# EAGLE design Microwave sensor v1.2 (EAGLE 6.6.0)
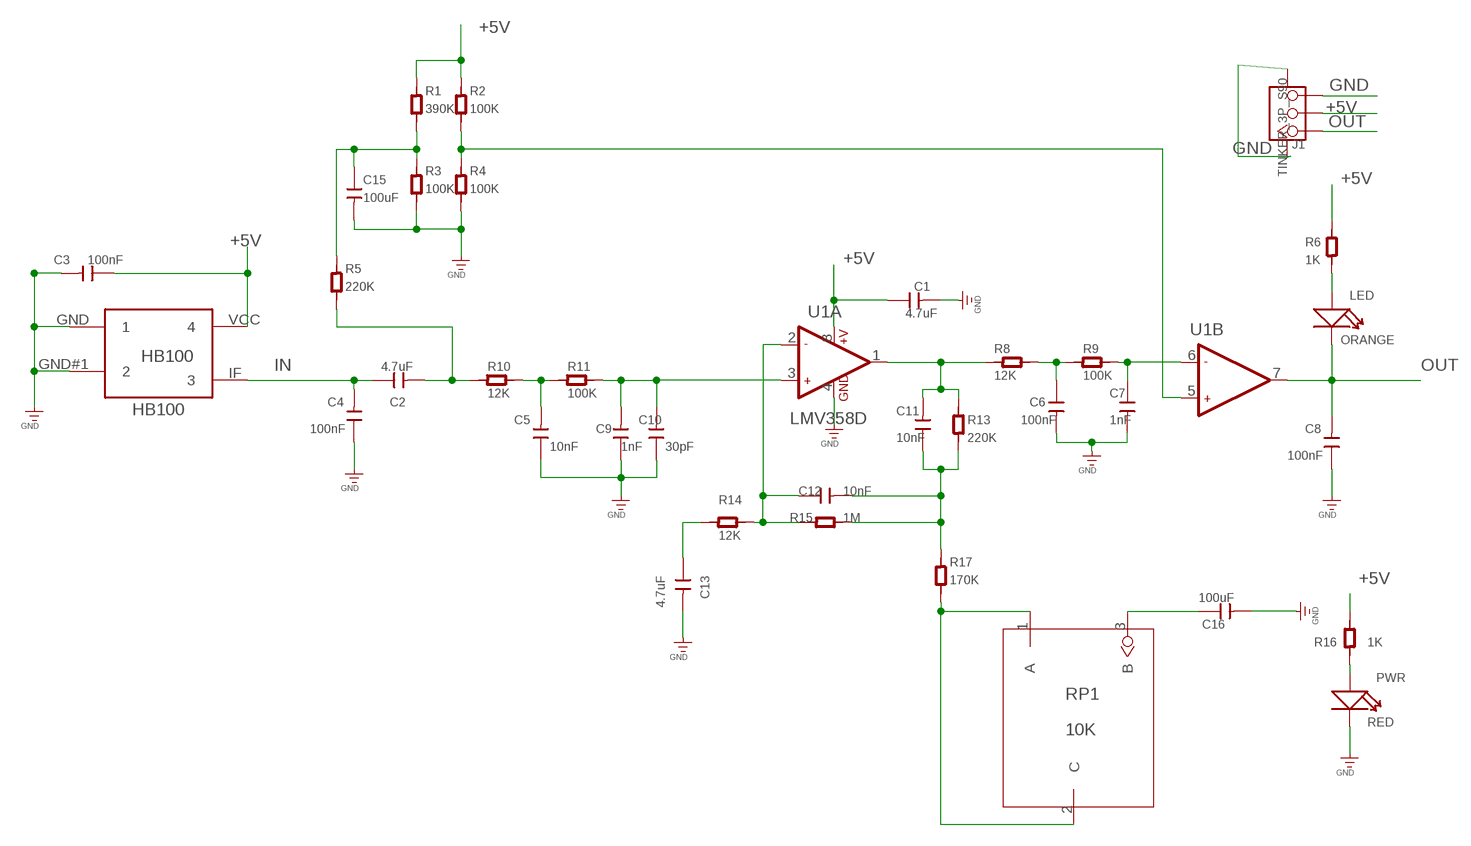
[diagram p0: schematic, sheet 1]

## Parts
C1  4.7uF  C-0603  [C0603]
C2  4.7uF  C-0603  [C0603]
C3  100nF  C-0603  [C0603]
C4  100nF  C-0603  [C0603]
C5  10nF  C-0603  [C0603]
C6  100nF  C-0603  [C0603]
C7  1nF  C-0603  [C0603]
C8  100nF  C-0603  [C0603]
C9  1nF  C-0603  [C0603]
C10  30pF  C-0603  [C0603]
C11  10nF  C-0603  [C0603]
C12  10nF  C-0603  [C0603]
C13  4.7uF  C-0603  [C0603]
C15  100uF  C-1210  [C1210]
C16  100uF  C-1210  [C1210]
HB100  MICROWAVE  [MICROWAVE]
J1  TINKER_3P_S90  [TINKER_3P_S90]
LED  ORANGE  LED'0805'  [LED-0805]
PWR  RED  LED'0805'  [LED-0805]
R1  390K  R-0603  [R0603]
R2  100K  R-0603  [R0603]
R3  100K  R-0603  [R0603]
R4  100K  R-0603  [R0603]
R5  220K  R-0603  [R0603]
R6  1K  R-0603  [R0603]
R8  12K  R-0603  [R0603]
R9  100K  R-0603  [R0603]
R10  12K  R-0603  [R0603]
R11  100K  R-0603  [R0603]
R13  220K  R-0603  [R0603]
R14  12K  R-0603  [R0603]
R15  1M  R-0603  [R0603]
R16  1K  R-0603  [R0603]
R17  170K  R-0603  [R0603]
RP1  10K  DEVICE_RESISTANCE  [PACKAGE__RESISTANCE]
U1  LMV358D  [SO08]

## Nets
+5V: C1.1 C3.1 HB100.VCC J1.2 R1.1 R2.1 R6.2 R16.2 U1.8(A:+V)
GND: C1.2 C3.2 C4.1 C5.1 C6.2 C7.2 C8.1 C9.1 C10.1 C13.2 C15.2 C16.2 HB100.GND HB100.GND#1 J1.3 J1.SS1 J1.SS2 PWR.- R3.2 R4.2 U1.4(A:GND)
IN: C2.1 C4.2 HB100.IF
N$1: C15.1 R1.2 R3.1 R5.1
N$3: C6.1 R8.2 R9.1
N$4: R2.2 R4.1 U1.5(B:+IN2)
N$5: C13.1 R14.1
N$6: C2.2 R5.2 R10.1
N$7: C11.1 C12.2 R13.1 R15.2 R17.1
N$8: C5.2 R10.2 R11.1
N$9: C11.2 R8.1 R13.2 U1.1(A:OUT1)
N$10: C9.2 C10.2 R11.2 U1.3(A:+IN1)
N$11: C7.1 R9.2 U1.6(B:-IN2)
N$12: C12.1 R14.2 R15.1 U1.2(A:-IN1)
N$13: R17.2 RP1.1(A) RP1.2(C)
N$14: C16.1 RP1.3(B)
N$16: PWR.+ R16.1
N$17: LED.+ R6.1
OUT: C8.2 J1.1 LED.- U1.7(B:OUT2)

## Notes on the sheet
- HB100

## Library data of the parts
C1-C13 C15 C16 = Discrete:C*: Ceramic Capacitors
HB100 = Microwave:MICROWAVE
J1 = Connector:TINKER_3P_S90
LED PWR = Discrete:LED*
R1-R6 R8-R11 R13-R17 = OPL Eagle Library:R*
RP1 = test:DEVICE_RESISTANCE
U1 = IC:LMV358: General purpose LOW Voltage, Rail-to-Rail Output Amplifiers http://www.fairchildsemi.com/ds/LM/LMV358.pdf

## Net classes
0 default: width 0.152 mm, drill 0.305 mm, clearance 0.152 mm

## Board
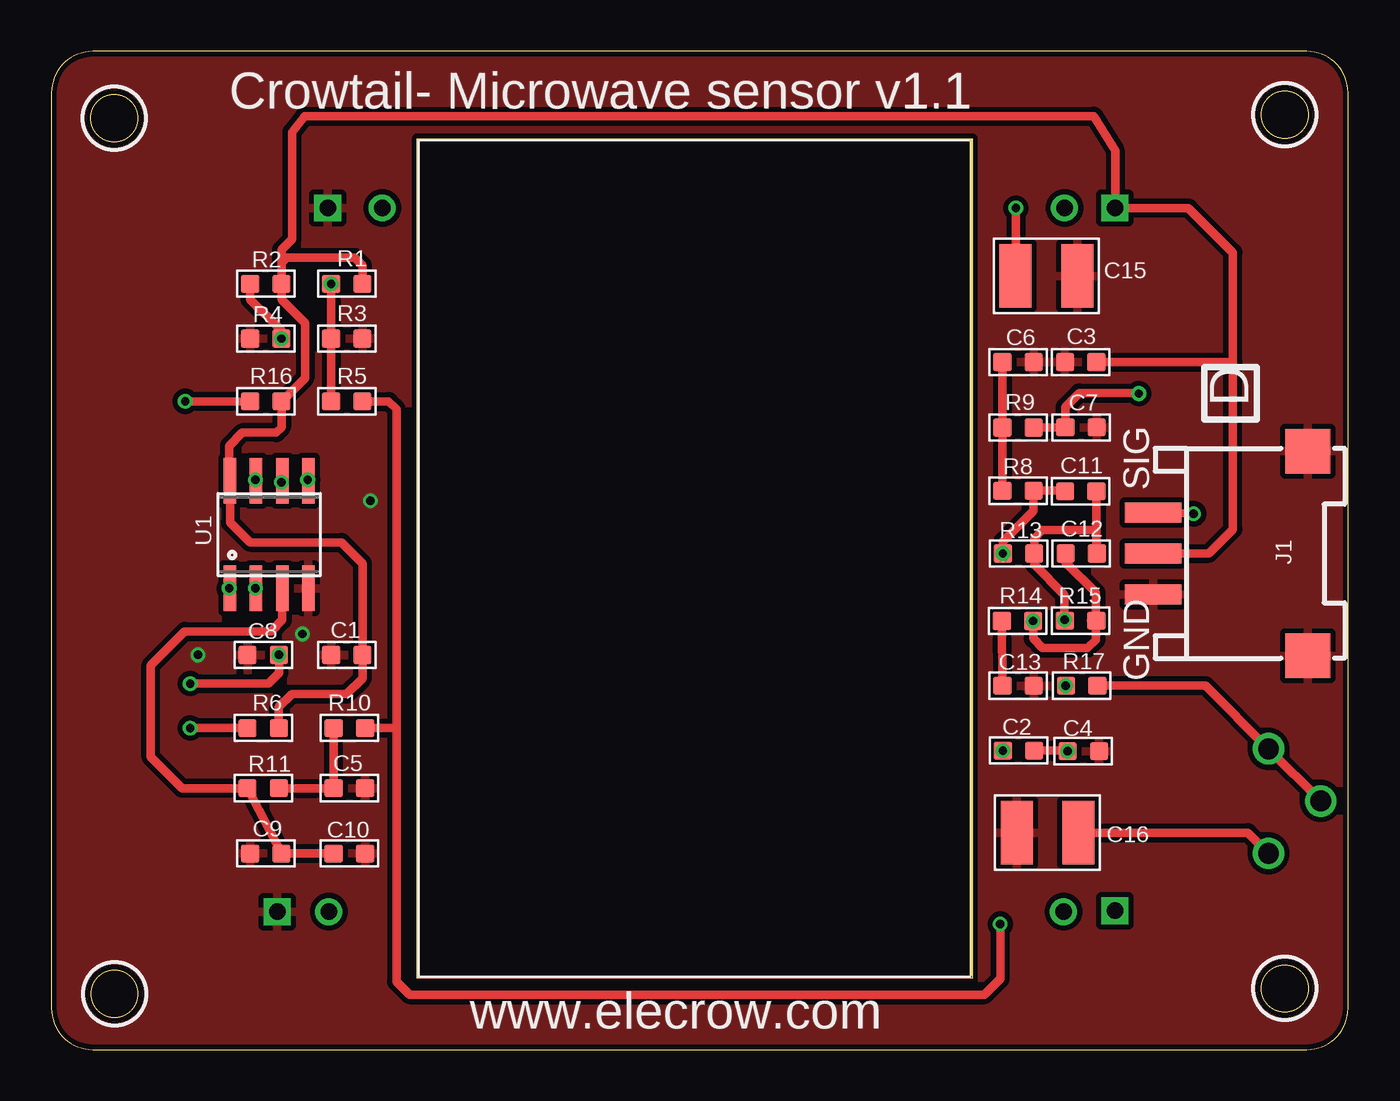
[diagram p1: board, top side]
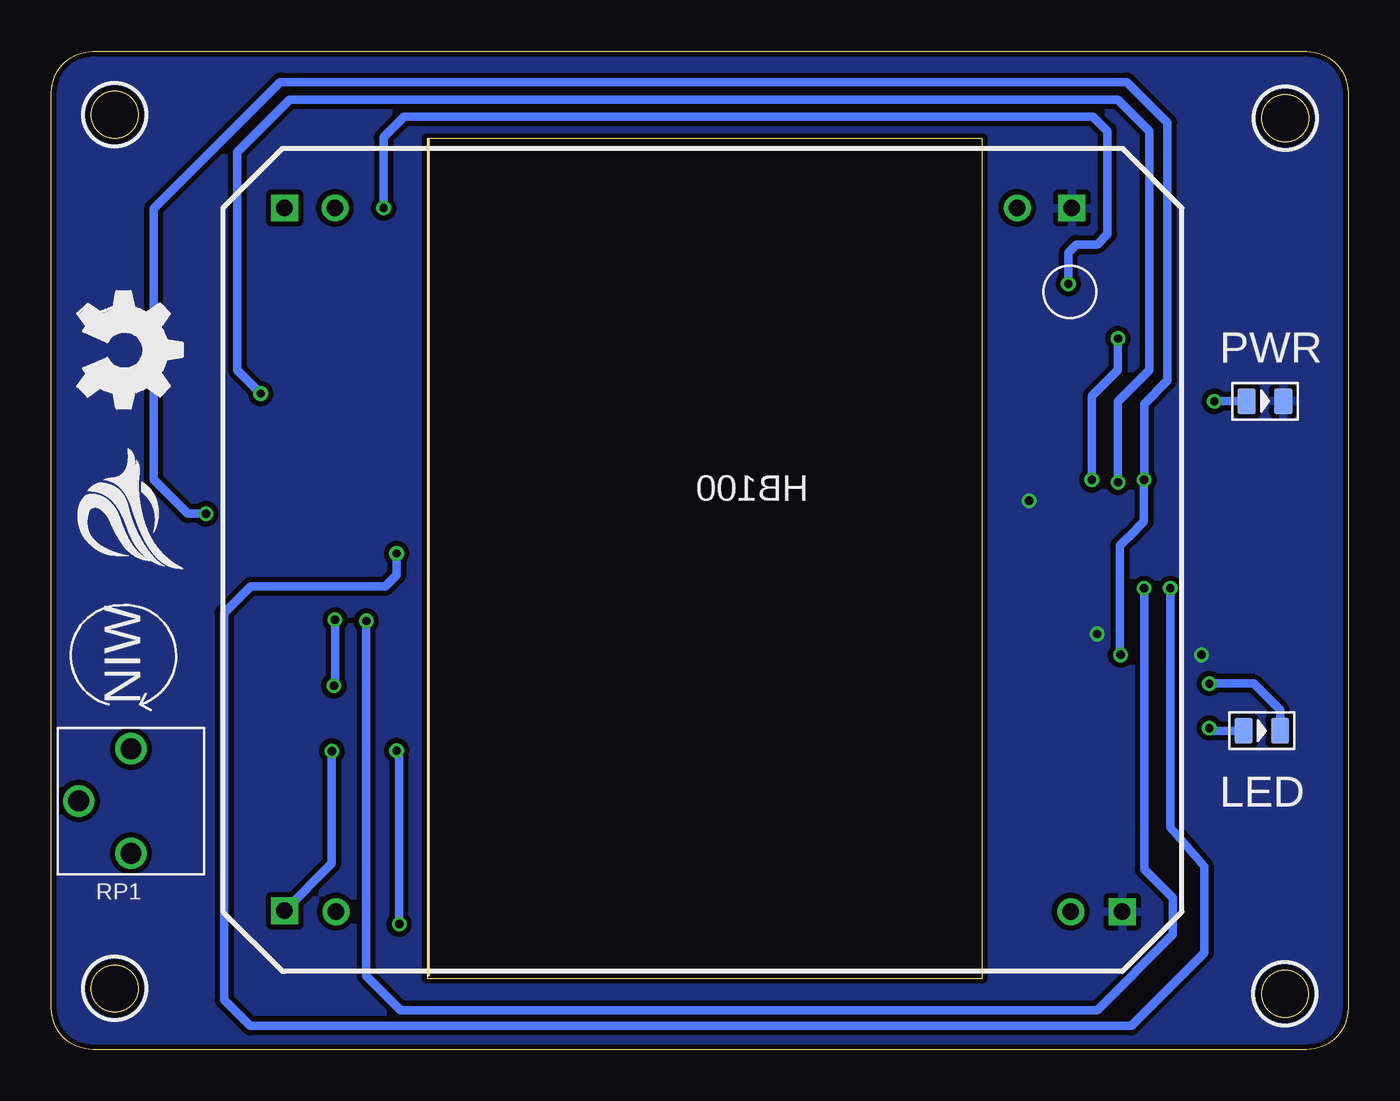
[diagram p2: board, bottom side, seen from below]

Size 63 x 48.5 mm. Coordinates in mm from the lower left corner, seen from the top.
Outline: 0,46.5 0,2 arc90 2,0 61,0 arc90 63,2 63,46.5 arc90 61,48.5 2,48.5 arc90 0,46.5
Outline: 17.75,44.27 44.76,44.27 44.76,3.45 17.75,3.45 17.75,44.27
Outline: circle at 3.06,2.71 radius 1.14
Outline: circle at 3.05,45.26 radius 1.14
Outline: circle at 59.92,45.42 radius 1.14
Outline: circle at 59.92,2.97 radius 1.14
Copper layers (1*16): Top 0.035mm / dielectric 1.5mm / Bottom 0.035mm
Design rules: minimum track width 6mil, minimum drill 12mil, track to track 6mil, track to pad 6mil, pad to pad 6mil, via to via 6mil, smd to smd 0mil, copper to edge 10mil, drill to drill 10mil, minimum pad ring 10mil, minimum via ring 6mil, stop-mask expansion 2mil, vias tented up to drill 100mil, thermal gap 10mil

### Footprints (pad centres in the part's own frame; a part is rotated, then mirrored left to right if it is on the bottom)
C0603 = smd 0.889 x 0.889: 1 -0.762,0; 2 0.762,0
C1210 = smd 1.55 x 3.1: 1 -1.5,0; 2 1.5,0
MICROWAVE = drill 0.8 square: GND 2.45,37.1; GND#1 0,2.9; IF 40.7,2.95; VCC 40.7,37.1 | drill 0.8: P$2 2.5,2.9; P$4 38.2,2.9; P$6 5.1,37.1; P$8 38.25,37.1
TINKER_3P_S90 = smd 0.965 x 2.74: 1 -1.984,-4.545; 2 0.016,-4.545; 3 2.016,-4.545 | smd 2.159 x 2.184: SS1 -4.958,2.955; SS2 4.99,2.955
LED-0805 = smd 0.889 x 1.27: + -0.889,0; - 0.889,0
R0603 = smd 0.889 x 0.889: 1 -0.762,0; 2 0.762,0
PACKAGE__RESISTANCE = drill 1.016: 1 -2.286,-0.254; 2 0.254,-2.794; 3 2.794,-0.254
SO08 = smd 0.61 x 2.21: 1 -1.905,-2.616; 2 -0.635,-2.616; 3 0.635,-2.616; 4 1.905,-2.616; 5 1.905,2.616; 6 0.635,2.616; 7 -0.635,2.616; 8 -1.905,2.616

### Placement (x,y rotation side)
C1  14.35,19.18 180 top
C2  46.99,14.53 180 top
C3  50.01,33.4 180 top
C4  50.14,14.5 180 top
C5  14.48,12.7 180 top
C6  46.96,33.4 0 top
C7  50.02,30.23 0 top
C8  10.29,19.18 0 top
C9  10.41,9.53 0 top
C10  14.48,9.53 180 top
C11  50.01,27.13 180 top
C12  50.04,24.1 0 top
C13  46.96,17.68 0 top
C15  48.35,37.59 0 top
C16  48.4,10.54 180 top
HB100  10.98,3.8 0 top
J1  58.08,24.12 270 top
LED  4.19,15.49 0 bottom
PWR  4.04,31.5 0 bottom
R1  14.35,37.21 180 top
R2  10.41,37.21 180 top
R3  14.35,34.54 0 top
R4  10.41,34.54 180 top
R5  14.35,31.5 0 top
R6  10.29,15.62 0 top
R8  46.96,27.15 180 top
R9  46.96,30.23 0 top
R10  14.48,15.62 180 top
R11  10.29,12.7 180 top
R13  46.99,24.1 180 top
R14  46.94,20.83 0 top
R15  50,20.83 180 top
R16  10.41,31.5 0 top
R17  50.06,17.68 0 top
RP1  58.88,12.33 270 bottom
U1  10.58,25.03 0 top
U$13  [ELECROW_NEW_4]  61.73,29.21 270 bottom
U$14  [OSHW_FILLX200_NOTEXT]  61.73,36.83 270 bottom
U$16  [MINIMUM]  63,16.51 0 bottom

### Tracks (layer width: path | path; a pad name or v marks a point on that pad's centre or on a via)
+5V
  Top 0.406: C3.1 57.4,33.4 | 11.18,38.23 R2.1 11.18,36.45 12.32,35.31 12.32,32.64 R16.2 11.18,30.23 10.92,29.97 9.27,29.97 8.64,29.34 8.64,27.68 U1.8 8.67,25.62 9.65,24.64 14.1,24.64 15.11,23.62 C1.1 15.11,18.03 14.35,17.27 11.68,17.27 11.05,16.64 R6.2 | 11.18,38.23 11.18,38.86 11.68,39.37 11.68,44.58 12.29,45.36 50.65,45.36 51.69,43.69 HB100.VCC 55.24,40.89 57.4,38.73 57.4,33.4 | R1.1 15.11,38.1 14.73,38.48 11.43,38.48 11.18,38.23 | J1.2 56.23,24.1 57.4,25.27 57.4,33.4
GND  (via drill 0.41)
  other vias: 15.49,26.67 12.19,20.19 7.11,19.18
  pour Bottom (isolate 0.254): -0.38,49.02 63.5,49.02 63.5,-0.38 -0.38,-0.38
  pour Top (isolate 0.254): -0.38,49.02 63.5,49.02 63.5,-0.38 -0.38,-0.38
IN  (via drill 0.41)
  Top 0.406: C2.1 49.34,14.53 C4.2
  Bottom 0.406: C4.2 49.38,9.05 HB100.IF
  other vias: 49.37,14.5
N$1  (via drill 0.41)
  Top 0.406: v46.86,40.89 46.86,37.61 C15.1 | R1.2 R3.1 R5.1
  Bottom 0.406: R1.2 13.59,38.73 13.21,39.12 12.19,39.12 11.68,39.62 11.68,44.63 12.39,45.34 45.85,45.34 46.86,44.33 v46.86,40.89
  other vias: 13.59,37.21
N$3
  Top 0.406: C6.1 R9.1 R8.2
N$4  (via drill 0.41)
  Top 0.406: R4.1 11.18,34.92 9.65,36.45 R2.2 | v12.45,27.69 v12.45,27.68 U1.5
  Bottom 0.406: R4.1 11.18,33.02 12.45,31.75 v12.45,27.69
  other vias: 11.18,34.54
N$5
  Top 0.406: R14.1 C13.1
N$6  (via drill 0.41)
  Top 0.406: R5.2 16.38,31.5 16.76,31.11 16.76,15.62 | 16.76,15.62 16.76,3.3 17.4,2.67 45.34,2.67 46.1,3.43 v46.1,6.1 | R10.1 16.76,15.62
  Bottom 0.406: v46.1,6.1 46.1,14.22 C2.2
  other vias: 46.23,14.53
N$7  (via drill 0.41)
  Top 0.406: R15.2 v49.23,20.88 49.23,22.1 47.75,23.57 R13.1 47.75,24.84 48.16,25.25 50.77,25.25 | R17.1 v49.28,17.68 49.28,17.73 | C11.1 50.77,25.25 | 50.77,25.25 50.77,24.13 C12.2 50.8,24.59
  Bottom 0.406: v49.23,20.88 49.23,17.73 v49.28,17.68
N$8
  Top 0.406: R11.1 C5.2 R10.2
N$9  (via drill 0.41)
  Top 0.406: C11.2 49,27.15 R8.1 47.7,27.13 47.7,26.16 46.23,24.69 R13.2 | U1.1 v8.64,22.41
  Bottom 0.406: v8.64,22.41 8.64,10.79 6.99,8.89 6.99,4.7 10.54,1.14 53.34,1.14 54.61,2.41 54.61,21.21 53.31,22.5 46.79,22.5 46.23,23.06 R13.2
  other vias: 46.23,24.1
N$10
  Top 0.406: U1.3 11.21,20.86 10.67,20.32 6.48,20.32 4.83,18.67 4.83,14.22 6.35,12.7 R11.2 C9.2 C10.2
N$11  (via drill 0.41)
  Top 0.406: U1.6 v11.18,27.56 | 49.02,30.32 C7.1 | R9.2 C7.1 | C7.1 49.26,31.23 49.94,31.9 52.81,31.9 v52.83,31.88
  Bottom 0.406: v11.18,27.56 11.18,31.5 9.65,33.02 9.65,44.63 11.18,46.15 51.44,46.15 53.98,43.61 53.98,33.02 v52.83,31.88
N$12  (via drill 0.41)
  Top 0.406: U1.2 v9.91,22.41 | 50.52,20.82 R15.1 | 50.49,20.85 R15.1 | R14.2 47.7,19.96 48.16,19.51 50.34,19.51 50.75,19.91 50.75,20.82 R15.1 | C12.1 49.28,23.67 50.75,22.2 50.75,20.85 R15.1
  Bottom 0.406: v9.91,22.41 9.91,8.76 8.51,7.37 8.51,5.59 12.19,1.91 46.02,1.91 47.7,3.58 R14.2
  other vias: 47.7,20.83
N$13
  Top 0.406: R17.2 56.07,17.68 RP1.1 RP1.2
N$14
  Top 0.406: C16.1 58.13,10.54 RP1.3
N$16  (via drill 0.41)
  Top 0.406: R16.1 v6.5,31.5
  Bottom 0.406: v6.5,31.5 PWR.+
N$17  (via drill 0.41)
  Top 0.406: R6.1 v6.74,15.62
  Bottom 0.406: LED.+ 6.74,15.49 v6.74,15.62
OUT  (via drill 0.41)
  Top 0.406: U1.7 v9.91,27.69 | J1.1 v55.5,26.04 | v6.74,17.78 10.55,17.78 11.06,18.29 C8.2
  Bottom 0.406: v55.5,26.04 56.39,26.04 58.04,27.69 58.04,40.87 51.89,47.02 10.74,47.02 8.77,45.04 8.77,32.51 9.91,31.38 v9.91,27.69 9.91,25.65 10.68,24.89 10.71,24.89 11.1,24.5 11.1,19.23 C8.2 | LED.- 3.3,16.5 4.58,17.78 v6.74,17.78
  other vias: 11.05,19.18

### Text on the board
tPlace: Crowtail- Microwave sensor v1.1 | D | SIG | GND | www.elecrow.com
